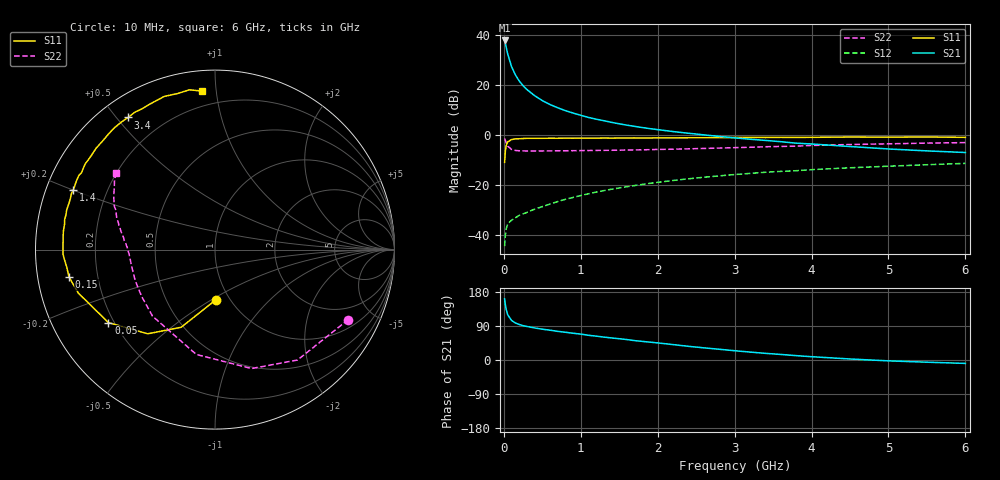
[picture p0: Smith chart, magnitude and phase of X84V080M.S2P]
! SIEMENS Small Signal Semiconductors
! BFP136W
! Si NPN RF Bipolar Junction Transistor in SOT343
! VCE = 4 V  IC = 80 mA
! Common Emitter S-Parameters:  September  1994
# GHz  S  MA  R  50
!  f  S11  S21  S12  S22
! GHz  MAG  ANG  MAG  ANG  MAG  ANG  MAG  ANG
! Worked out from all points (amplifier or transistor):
!   40 points, 10 MHz to 6 GHz, reference 50 ohm
!   highest |S21| = 37.7 dB at 10 MHz (marker M1)
!   |S21| within 3 dB of that: start of sweep to 32.98 MHz
!   unconditionally stable (mu >= 1): 603.1 MHz to 2.896 GHz
!   at 200 MHz: K = 0.63, MSG = 26.9 dB, |S12| = -32.3 dB
!   at 1.5 GHz: K = 1.10, MAG = 10.9 dB, |S12| = -21.3 dB
!   at 6 GHz: K = 0.97, MSG = 2.2 dB, |S12| = -11.5 dB
!   S11 on the Smith chart (normalised r, x): 10 MHz: 0.86, -0.52; 50 MHz: 0.18, -0.30; 150 MHz: 0.09, -0.09; 1.4 GHz: 0.08, +0.20; 3.4 GHz: 0.08, +0.54; 6 GHz: 0.11, +0.91
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0.01  0.2804 -89.2  76.89 161.3  0.0059 69.9  0.8385 -27.7
0.02  0.4716 -113.5  66.86 145.5  0.0098 60.4  0.7681 -53.2
0.03  0.6002 -128.6  57.11 133.9  0.013 51.0  0.6933 -72.9
0.05  0.7199 -145.6  41.37 119.5  0.0164 40.3  0.5934 -100.1
0.1  0.7992 -162.4  23.11 104.4  0.0195 35.5  0.5086 -133.2
0.15  0.828 -169.4  15.77 97.8  0.0218 37.5  0.4848 -147.4
0.2  0.8313 -173.1  11.87 93.7  0.0244 39.2  0.4778 -155.2
0.25  0.8406 -176.2  9.577 90.7  0.0261 41.9  0.4756 -160.2
0.3  0.8471 -178.2  8.015 88.5  0.028 43.7  0.4735 -163.6
0.4  0.8471 177.9  6.041 84.6  0.0324 47.9  0.4735 -168.1
0.5  0.8492 175.0  4.819 81.3  0.0365 50.8  0.4741 -171.2
0.6  0.8509 173.0  4.02 78.7  0.0411 53.0  0.4752 -173.1
0.7  0.8501 170.4  3.465 75.6  0.046 55.5  0.4769 -174.5
0.9  0.8528 166.8  2.713 70.6  0.0557 57.4  0.4793 -177.2
1.1  0.8534 162.3  2.218 65.2  0.0658 58.3  0.4834 -178.9
1.4  0.8562 157.3  1.769 58.3  0.0813 58.6  0.4886 178.8
2.2  0.8653 143.3  1.158 40.6  0.1215 54.4  0.5132 172.7
3.2  0.8816 126.4  0.813 20.9  0.1684 45.6  0.5614 164.0
3.4  0.8811 123.3  0.77 17.6  0.1776 43.6  0.5751 162.2
4.5  0.8992 108.3  0.581 2.7  0.2183 33.6  0.6374 152.3
5.5  0.9016 99.1  0.475 -5.8  0.2512 25.9  0.6801 145.4
6  0.8863 94.8  0.441 -9.0  0.2674 21.6  0.6963 142.4
